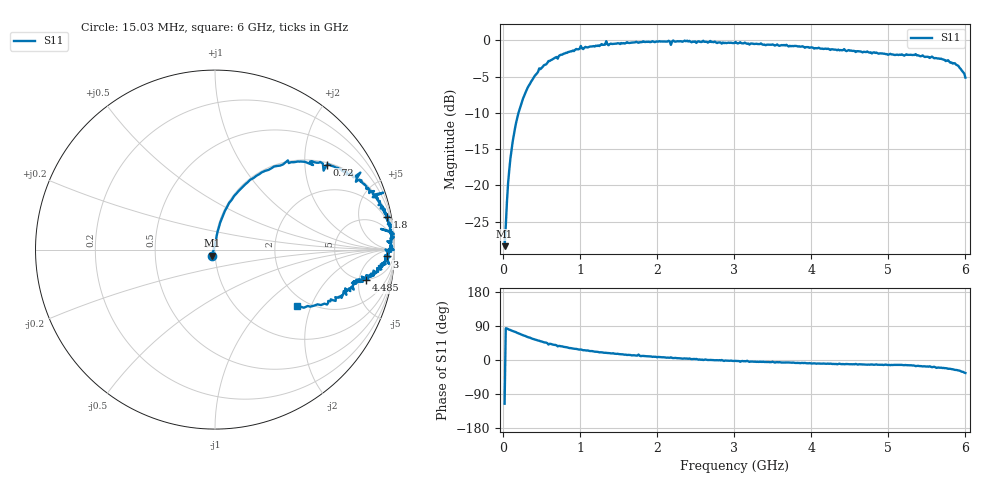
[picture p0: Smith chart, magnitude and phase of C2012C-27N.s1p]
!	Network	Analyzer	HP8753E.07.74:	Oct	30	2002	Serial	No.	JP38451487
!	Hewlett-Packard
!	7	Sep	2009	10:49:08
!	Frequency	S11
#	HZ	S	RI	R	50
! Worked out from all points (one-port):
!   400 points, 15.03 MHz to 6 GHz, reference 50 ohm
!   lowest |S11| = -28.4 dB at 15.03 MHz (marker M1), VSWR 1.08, Z = 48.3 - j3.33 ohm
!   |S11| at or under -10 dB: start of sweep to 195 MHz
!   S11 on the Smith chart (normalised r, x): 15.03 MHz: 0.97, -0.07; 720 MHz: 1.06, +2.59; 1.8 GHz: 1, +10; 3 GHz: 25, -24; 4.485 GHz: 4.87, -6.28; 6 GHz: 1.77, -1.60
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1.502992e7  -0.0163 -0.0344
6.00297e7  0.0149 0.102
9.002955e7  0.0287 0.15
1.95029e8  0.106 0.298
4.650277e8  0.406 0.497
7.200264e8  0.623 0.473
7.650262e8  0.646 0.468
1.005025e9  0.81 0.429
1.320023e9  0.885 0.306
1.335023e9  0.937 0.317
1.365023e9  0.879 0.292
1.515022e9  0.911 0.248
1.725021e9  0.959 0.197
1.755021e9  0.933 0.24
1.800021e9  0.957 0.182
2.145019e9  0.989 0.107
2.175019e9  0.925 0.115
2.205019e9  0.996 0.0872
2.265019e9  0.985 0.0836
3.000015e9  0.959 -0.0384
3.015015e9  0.975 -0.0402
3.765011e9  0.907 -0.107
4.485008e9  0.841 -0.17
4.515007e9  0.837 -0.163
5.265004e9  0.773 -0.19
5.775001e9  0.672 -0.286
5.91e9  0.59 -0.309
6e9  0.458 -0.312
